PROGRAM MAIN
VAR
	m_Output1 AT%QX0.0 :BOOL;
	m_Output2 AT%QX0.1 :BOOL;
	m_Output3 AT%QX0.2 :BOOL;
	m_Output4 AT%QX0.3 :BOOL;
	m_Output5 AT%QX0.4 :BOOL;
	IntTest,IntTest2 :INT;
	DintTest:dint;
	RealTest,RealWriteOnly :REAL;
	LRealTest:LREAL;
	StringTest:string:='This is tc3_remote,do you copy?';
END_VAR

IF IntTest <32767 THEN
	IntTest := IntTest +1;
ELSE
		IntTest := -32768;
END_IF
IF GVL_IO.IntTest1 <32767 THEN
	GVL_IO.IntTest1:= GVL_IO.IntTest1 +10;
ELSE
	GVL_IO.IntTest1 := -32768;	
END_IF
IF IntTest2 <32767 THEN
	IntTest2 := IntTest2 +100;
ELSE
		IntTest2 := -32768;
END_IF

END_PROGRAM
